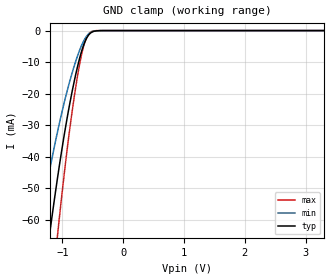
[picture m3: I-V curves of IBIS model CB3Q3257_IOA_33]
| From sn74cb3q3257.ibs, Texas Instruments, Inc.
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[Model]   CB3Q3257_IOA_33
Model_type  Terminator
| variable   typ   min   max
C_comp   5.19pF   3.43pF   9.55pF
| C_tri-state   5.19pF   3.43pF   9.55pF
[Temperature Range]   40   100   -40
| Ambient temperature   25   85   -40
[Voltage range]   3.3   3   3.6
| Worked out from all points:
|   GND clamp passes 1 mA (typ) near -0.55 V on its own axis
[GND Clamp]
| CB3Q3257_IOA_33
|   Voltage   I(typ)   I(min)   I(max)
-5.5V     -936.3mA   -734.9mA   -1.142A
-1.415V   -95.75mA   -66.13mA   -132.7mA
-1.365V   -87.81mA   -60.53mA   -121.9mA
-1.215V   -65.19mA   -44.76mA   -90.88mA
-1.19V    -61.61mA   -42.29mA   -85.89mA
-1.085V   -47.29mA   -32.47mA   -65.73mA
-1.065V   -44.7mA    -30.7mA    -62.04mA
-920mV    -27.46mA   -18.98mA   -37.35mA
-760mV    -12.12mA   -8.508mA   -15.39mA
-645mV    -4.293mA   -3.108mA   -4.499mA
-545mV    -907uA     -714.8uA   -587.9uA
3.3V      197.8pA    862.6pA    19.5pA
